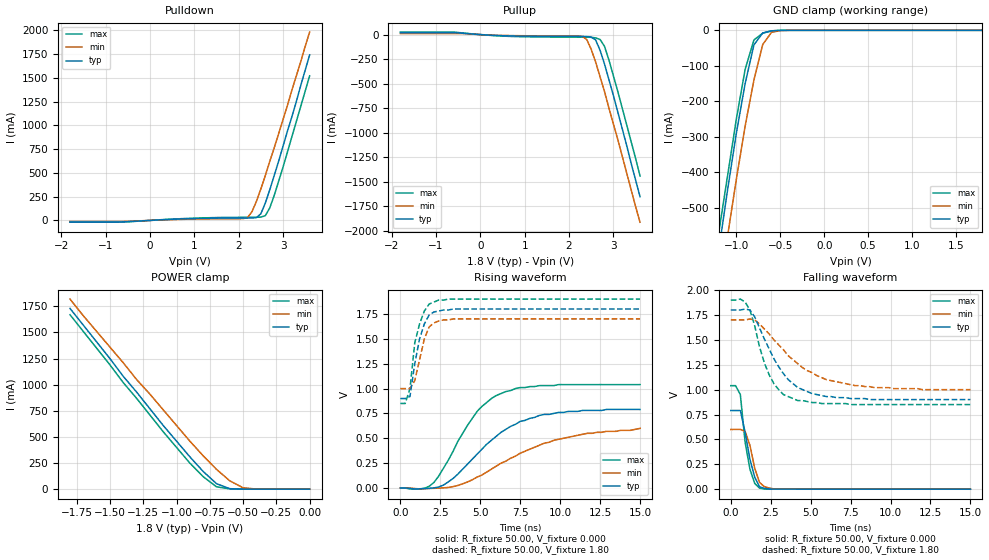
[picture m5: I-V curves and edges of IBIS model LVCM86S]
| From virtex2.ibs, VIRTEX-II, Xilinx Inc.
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|   Model LVCM86S
[Model]   LVCM86S
Model_type   I/O
Polarity   Non-Inverting
Enable   Active-Low
Vinh = 1.19V
Vinl = 0.4V
Vmeas =   0.90V
Cref =  35.00pF
Rref =   1.00M
Vref =  0.000V
C_comp   7.00pF   6.00pF   8.00pF
[Temperature Range]   25.00   100.00   0.000
[Voltage Range]   1.80V   1.70V   1.90V
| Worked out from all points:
|   slope of the pulldown table from 0 to 0.27 V, typ, clamps not added: 40.1 ohm
|   slope of the pullup table from 0 to 0.27 V, typ, clamps not added: 38.7 ohm
|   GND clamp passes 1 mA (typ) near -0.57 V on its own axis
|   POWER clamp passes 1 mA (typ) near -0.52 V on its own axis
|   rising waveform, R_fixture 50.00, V_fixture 0.000: 20-80 % time 3.37ns typ, 4.65ns min, 2.46ns max; typ from 0 V to 0.79 V
|   rising waveform, R_fixture 50.00, V_fixture 1.80: 20-80 % time 695ps typ, 664ps min, 653ps max; typ from 0.9 V to 1.8 V
|   falling waveform, R_fixture 50.00, V_fixture 0.000: 20-80 % time 621ps typ, 576ps min, 517ps max; typ from 0.79 V to 0 V
|   falling waveform, R_fixture 50.00, V_fixture 1.80: 20-80 % time 1.95ns typ, 3ns min, 1.29ns max; typ from 1.8 V to 0.9 V
[Pulldown]
| voltage   I(typ)   I(min)   I(max)
-1.8V     -16.21mA   -10.88mA   -18.68mA
-700mV    -16.21mA   -10.88mA   -18.68mA
900mV     18.14mA    13.2mA     21.9mA
2.2V      25.3mA     29.45mA    32.42mA
2.3V      25.57mA    91.27mA    32.53mA
2.4V      28.85mA    200mA      32.79mA
2.5V      69.55mA    330mA      34.56mA
2.6V      180mA      470mA      49.6mA
2.7V      320mA      620mA      130mA
2.8V      470mA      760mA      260mA
3V        780mA      1.06A      560mA
3.6V      1.74A      1.98A      1.52A
[Pullup]
| voltage   I(typ)   I(min)   I(max)
-1.8V     19.87mA    11.13mA    25.49mA
-600mV    19.87mA    11.13mA    25.49mA
600mV     -12.68mA   -9.53mA    -17.16mA
2.2V      -18.23mA   -14.18mA   -25.95mA
2.3V      -18.43mA   -18.65mA   -26.1mA
2.4V      -19.61mA   -50.36mA   -26.33mA
2.5V      -25.25mA   -150mA     -27.63mA
2.6V      -54.62mA   -280mA     -33.58mA
2.7V      -160mA     -430mA     -50.04mA
2.8V      -300mA     -580mA     -120mA
3.1V      -790mA     -1.07A     -580mA
3.6V      -1.65A     -1.91A     -1.44A
[GND_clamp]
| voltage   I(typ)   I(min)   I(max)
-1.8V     -1.65A     -1.74A     -1.6A
-1.2V     -620mA     -740mA     -570mA
-1.1V     -450mA     -580mA     -410mA
-1V       -290mA     -420mA     -250mA
-900mV    -150mA     -270mA     -110mA
-800mV    -40.97mA   -140mA     -27.17mA
-700mV    -7.54mA    -40.17mA   -8.08mA
-600mV    -1.39mA    -5.57mA    -1.57mA
-500mV    -120uA     -660uA     -120uA
1.8V      34.27pA    98.88nA    22.46pA
[POWER_clamp]
| voltage   I(typ)   I(min)   I(max)
-1.8V     1.73A      1.82A      1.67A
-1.7V     1.57A      1.66A      1.51A
-1.4V     1.08A      1.21A      1.02A
-1.3V     930mA      1.05A      870mA
-1.1V     610mA      760mA      550mA
-900mV    310mA      460mA      250mA
-800mV    170mA      320mA      120mA
-700mV    52.75mA    190mA      22.81mA
-600mV    4.57mA     79.88mA    2.44mA
-500mV    270uA      13.45mA    250uA
-400mV    16.38uA    820uA      14.46uA
0V        34.27pA    1.07nA     29.84pA
[Ramp]
| variable   typ   min   max
dV/dt_r   0.47/3.34n   0.35/4.50n   0.63/2.45n
dV/dt_f   0.54/1.98n   0.42/3.02n   0.63/1.34n
R_load = 50.00
[Rising Waveform]
R_fixture = 50.00
V_fixture = 0.000
| time   V(typ)   V(min)   V(max)
0s        0V         0V         0V
1.5ns     -6.08mV    -6.55mV    -3.07mV
2.1ns     1.12mV     -2.82mV    56.19mV
3.3ns     96.24mV    14.05mV    370mV
4.8ns     340mV      110mV      770mV
6ns       520mV      220mV      930mV
7.5ns     670mV      350mV      1.01V
9ns       740mV      450mV      1.03V
11.7ns    780mV      550mV      1.04V
15ns      790mV      600mV      1.04V
[Rising Waveform]
R_fixture = 50.00
V_fixture = 1.80
V_fixture_min = 1.70
V_fixture_max = 1.90
| time   V(typ)   V(min)   V(max)
0s        900mV      1V         850mV
300ps     900mV      1V         850mV
600ps     920mV      1V         1V
900ps     1.25V      1.08V      1.46V
1.2ns     1.5V       1.29V      1.65V
1.5ns     1.65V      1.5V       1.78V
1.8ns     1.74V      1.62V      1.85V
2.4ns     1.78V      1.68V      1.89V
3.3ns     1.8V       1.7V       1.9V
15ns      1.8V       1.7V       1.9V
[Falling Waveform]
R_fixture = 50.00
V_fixture = 0.000
| time   V(typ)   V(min)   V(max)
0s        790mV      600mV      1.04V
300ps     790mV      600mV      1.04V
600ps     790mV      600mV      950mV
900ps     570mV      580mV      470mV
1.2ns     300mV      440mV      200mV
1.5ns     120mV      210mV      57.56mV
1.8ns     24.04mV    67.88mV    10.66mV
2.1ns     8.56mV     25.12mV    890uV
2.7ns     610uV      2.64mV     940uV
15ns      8.53uV     79.98uV    -51.27uV
[Falling Waveform]
R_fixture = 50.00
V_fixture = 1.80
V_fixture_min = 1.70
V_fixture_max = 1.90
| time   V(typ)   V(min)   V(max)
0s        1.8V       1.7V       1.9V
600ps     1.8V       1.7V       1.91V
1.2ns     1.8V       1.71V      1.8V
2.1ns     1.51V      1.61V      1.27V
2.7ns     1.31V      1.5V       1.06V
3.3ns     1.16V      1.4V       950mV
4.2ns     1.02V      1.26V      890mV
6ns       930mV      1.1V       860mV
9ns       900mV      1.02V      850mV
15ns      900mV      1V         850mV
